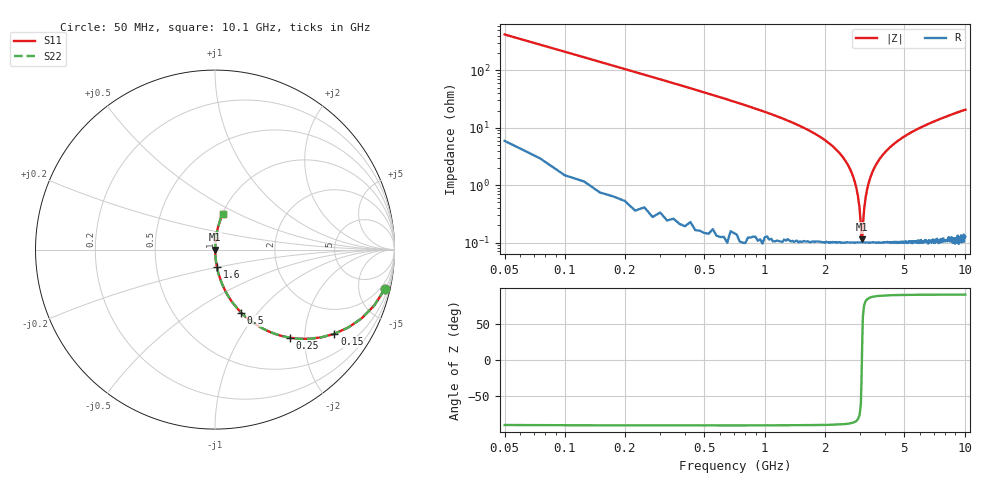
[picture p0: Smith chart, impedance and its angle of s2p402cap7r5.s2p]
! AVX Thin Film Operation		Date: April 2003
! Description: Accu-P® Series, Thin Film, SMD, RF Capacitor
! Part Number: 0402ZK7R5BBW
! 50 MHz  -  10.05 GHz
! Serial Measurements
# hz S db R 50
!	S11		S21		S12		S22
!	dB	Phase	dB	Phase	dB	Phase	dB	Phase
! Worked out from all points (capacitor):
!   400 points, 50 MHz to 10.1 GHz, reference 50 ohm
!   read as one part in series: C = 7.5 pF near 100 MHz
!   lowest |Z| = 114 mohm at 3.08 GHz (marker M1)
!   series resonance near 3.066 GHz, so ESL is about 360 pH
!   S11 on the Smith chart (normalised r, x): 50 MHz: 1.13, -8.50; 150 MHz: 1.02, -2.82; 250 MHz: 1.01, -1.69; 500 MHz: 1.00, -0.83; 1.6 GHz: 1.00, -0.19; 10.1 GHz: 1.00, +0.41
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5e7  -0.26 -13.2  -12.80 76.0  -12.80 76.0  -0.26 -13.2
1.5e8  -1.79 -35.2  -4.78 54.5  -4.78 54.5  -1.79 -35.2
2.5e8  -3.83 -49.7  -2.35 40.0  -2.35 40.0  -3.83 -49.7
5e8  -8.37 -67.4  -0.70 22.4  -0.70 22.4  -8.37 -67.4
1.6e9  -20.40 -83.9  -0.05 5.5  -0.05 5.5  -20.40 -83.9
1.73e9  -21.60 -84.5  -0.04 4.8  -0.04 4.8  -21.60 -84.5
2.43e9  -29.70 -86.4  -0.01 1.9  -0.01 1.9  -29.70 -86.4
2.73e9  -35.80 -85.5  -0.01 0.9  -0.01 0.9  -35.80 -85.5
2.93e9  -43.80 -80.7  -0.01 0.4  -0.01 0.4  -43.80 -80.7
2.98e9  -47.60 -75.9  -0.01 0.2  -0.01 0.2  -47.60 -75.9
3.03e9  -54.00 -59.8  -0.01 0.1  -0.01 0.1  -54.00 -59.8
3.05e9  -58.70 -30.4  -0.01 0.0  -0.01 0.0  -58.70 -30.4
3.08e9  -58.90 28.5  -0.01 -0.0  -0.01 -0.0  -58.90 28.5
3.1e9  -54.20 58.9  -0.01 -0.1  -0.01 -0.1  -54.20 58.9
3.15e9  -47.90 75.3  -0.01 -0.2  -0.01 -0.2  -47.90 75.3
3.2e9  -44.20 80.3  -0.01 -0.3  -0.01 -0.3  -44.20 80.3
3.4e9  -36.80 85.2  -0.01 -0.8  -0.01 -0.8  -36.80 85.2
4e9  -28.50 86.3  -0.01 -2.1  -0.01 -2.1  -28.50 86.3
5.08e9  -22.80 85.0  -0.03 -4.2  -0.03 -4.2  -22.80 85.0
6.75e9  -18.40 82.6  -0.07 -6.9  -0.07 -6.9  -18.40 82.6
8.43e9  -15.80 80.2  -0.13 -9.4  -0.13 -9.4  -15.80 80.2
1.01e10  -13.90 78.0  -0.19 -11.6  -0.19 -11.6  -13.90 78.0
